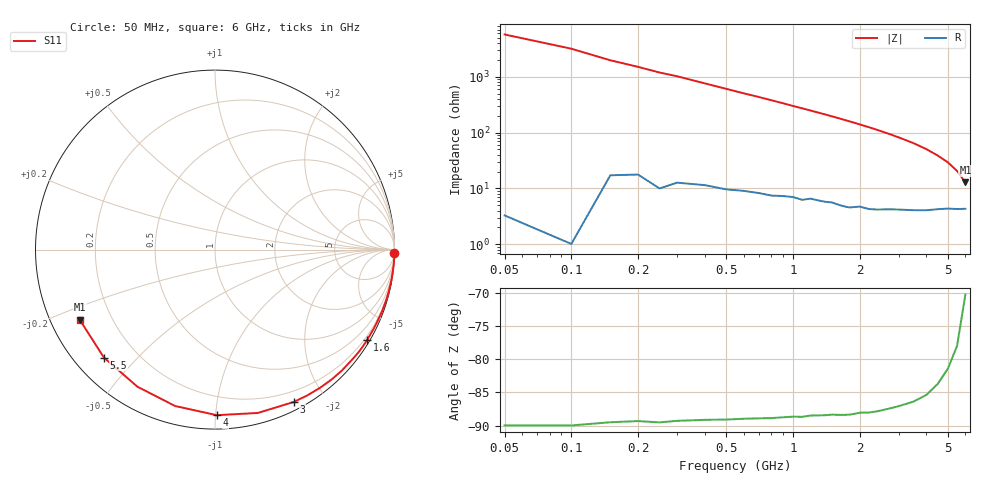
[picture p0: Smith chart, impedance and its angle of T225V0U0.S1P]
! SIEMENS Discrete & RF Semiconductors
! BAS70-04W
! Si Schottky Diode in SOT323
! VR = 25 V
! S-Parameters:  November  1997
# GHz  S  MA  R  50
!  f  S11
! GHz  MAG  ANG
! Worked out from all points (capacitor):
!   34 points, 50 MHz to 6 GHz, reference 50 ohm
!   read as one part to ground: C = 537 fF near 50 MHz
!   lowest |Z| = 12.8 ohm at 6 GHz (marker M1)
!   S11 on the Smith chart (normalised r, x): 50 MHz: open; 1.6 GHz: 0.10, -3.64; 3 GHz: 0.08, -1.64; 4 GHz: 0.08, -1.01; 5.5 GHz: 0.09, -0.40; 6 GHz: 0.09, -0.24
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0.05  1 -1.0
0.1  1 -1.8
0.15  0.9996 -2.9
0.25  0.9993 -4.8
0.3  0.9988 -5.6
0.4  0.998 -7.5
0.6  0.9965 -11.3
0.8  0.9949 -15.0
0.9  0.9937 -16.9
1  0.9925 -18.9
1.1  0.9919 -20.8
1.2  0.9899 -22.7
1.3  0.9889 -24.7
1.4  0.9879 -26.6
1.6  0.9858 -30.7
1.8  0.9837 -34.9
1.9  0.9815 -37.0
2.2  0.9767 -43.6
2.4  0.9726 -48.1
2.6  0.9671 -52.9
2.8  0.9614 -57.7
3  0.9558 -62.6
3.5  0.9409 -75.3
4  0.9225 -89.4
4.5  0.8993 -104.3
5  0.8778 -119.5
5.5  0.8631 -135.8
6  0.8491 -152.7
